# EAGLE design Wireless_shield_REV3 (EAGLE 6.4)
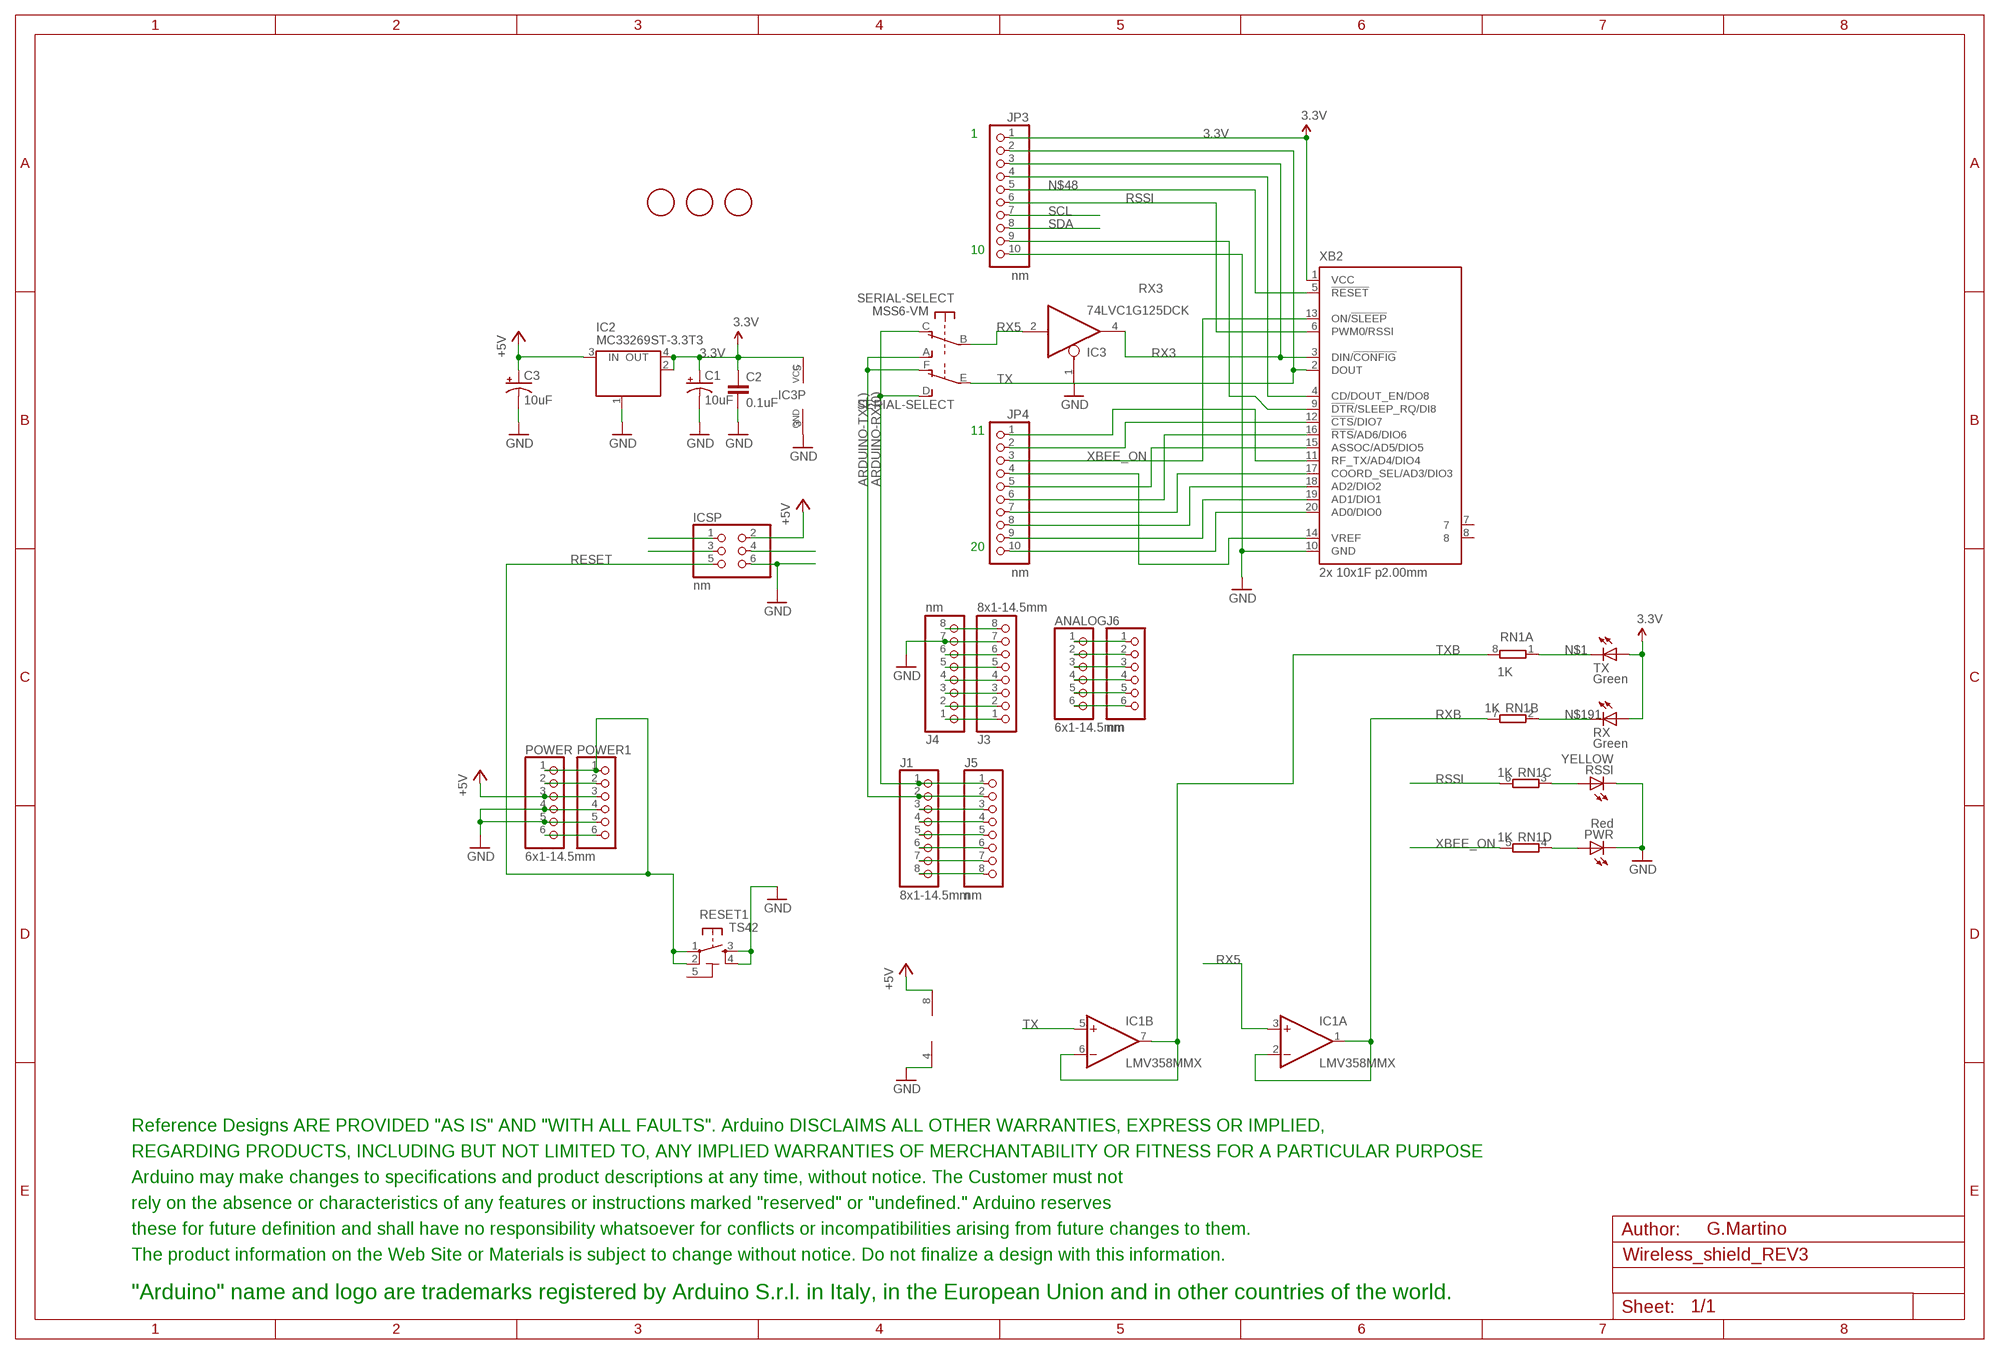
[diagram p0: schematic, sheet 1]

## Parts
A1  FIDUCIALMOUNT  [FIDUCIA-MOUNT]
A2  FIDUCIALMOUNT  [FIDUCIA-MOUNT]
A3  FIDUCIALMOUNT  [FIDUCIA-MOUNT]
ANALOG  6x1-14.5mm  PINHD-1X6  [1X06]
C1  10uF  CAP_POL1206  [EIA3216]
C2  0.1uF  CAP0603-CAP  [0603-CAP]
C3  10uF  CAP_POL1206  [EIA3216]
IC1  LMV358MMX  [MSOP08]
IC2  MC33269ST-3.3T3  [SOT223]
IC3  74LVC1G125DCK  [SC70-5]
ICSP  nm  PINHD-2X3  [2X03]
J1  8x1-14.5mm  PINHD-1X8  [1X08]
J3  8x1-14.5mm  PINHD-1X8  [1X08]
J4  nm  PINHD-1X8  [1X08]
J5  nm  PINHD-1X8  [1X08]
J6  nm  PINHD-1X6  [1X06]
JP3  nm  PINHD-1X10  [1X10]
JP4  nm  PINHD-1X10  [1X10]
POWER  6x1-14.5mm  PINHD-1X6  [1X06]
POWER1  PINHD-1X6  [1X06]
PWR  Red  LEDCHIP-LED0805  [CHIP-LED0805]
RESET1  TS42  [TS42]
RN1  1K  4R-NCAY16  [CAY16]
RSSI  YELLOW  LEDCHIP-LED0805  [CHIP-LED0805]
RX  Green  LEDCHIP-LED0805  [CHIP-LED0805]
SERIAL-SELECT  MSS6-VM  [MSS6-V]
TX  Green  LEDCHIP-LED0805  [CHIP-LED0805]
U$2  DISCLAIMER-SMALL  [DISCLAIMER]
XB2  2x 10x1F p2.00mm  XBEE-PRO  [XBEE-PRO]

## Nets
3.3V: C1.A(+) C2.1 IC2.2(OUT) IC2.4(OUT) IC3.5(VCC) JP3.1 RX.A TX.A XB2.1(VCC)
+5V: C3.A(+) IC1.8(P:V+) IC2.3(IN) ICSP.2 POWER1.3 POWER.3
ARDUINO-RX(0): J1.1 J5.1 SERIAL-SELECT.C(O) SERIAL-SELECT.D(S)
ARDUINO-TX(1): J1.2 J5.2 SERIAL-SELECT.A(S) SERIAL-SELECT.F(O)
GND: C1.C(-) C2.2 C3.C(-) IC1.4(P:V-) IC2.1(GND/ADJ) IC3.1(OE) IC3.3(GND) ICSP.6 J3.7 J4.7 JP3.10 POWER1.4 POWER1.5 POWER.4 POWER.5 PWR.C RESET1.3 RESET1.4 RSSI.C XB2.10(GND)
N$1: RN1.1 TX.C
N$2: J3.1 J4.1
N$3: ICSP.3
N$4: ICSP.1
N$5: ICSP.4
N$6: J3.2 J4.2
N$7: J3.3 J4.3
N$9: J3.6 J4.6
N$10: J1.3 J5.3
N$11: J1.4 J5.4
N$12: J1.5 J5.5
N$13: J1.6 J5.6
N$14: J1.7 J5.7
N$15: J1.8 J5.8
N$16: RN1.3 RSSI.A
N$18: ANALOG.1 J6.1
N$19: ANALOG.2 J6.2
N$20: ANALOG.3 J6.3
N$21: ANALOG.4 J6.4
N$22: ANALOG.5 J6.5
N$23: ANALOG.6 J6.6
N$24: JP4.10 XB2.20(AD0/DIO0)
N$25: JP4.9 XB2.19(AD1/DIO1)
N$27: J3.5 J4.5
N$28: JP4.8 XB2.18(AD2/DIO2)
N$29: PWR.A RN1.4
N$30: POWER1.6 POWER.6
N$33: JP4.7 XB2.17(COORD_SEL/AD3/DIO3)
N$34: JP4.6 XB2.16(!RTS!/AD6/DIO6)
N$36: JP4.5 XB2.15(ASSOC/AD5/DIO5)
N$37: JP4.4 XB2.14(VREF)
N$39: JP4.2 XB2.12(!CTS!/DIO7)
N$41: JP4.1 XB2.11(RF_TX/AD4/DIO4)
N$43: JP3.4 XB2.4(CD/DOUT_EN/DO8)
N$48: JP3.5 XB2.5(!RESET)
N$50: JP3.9 XB2.9(!DTR!/SLEEP_RQ/DI8)
N$61: J3.4 J4.4
N$191: RN1.2 RX.C
N$222: J3.8 J4.8
N$223: POWER1.2 POWER.2
RESET: ICSP.5 POWER1.1 POWER.1 RESET1.1 RESET1.2
RSSI: JP3.6 RN1.6 XB2.6(PWM0/RSSI)
RX3: IC3.4(O) JP3.3 XB2.3(DIN/!CONFIG)
RX5: IC1.3(A:+IN) IC3.2(I) SERIAL-SELECT.B(P)
RXB: IC1.1(A:OUT) IC1.2(A:-IN) RN1.7
SCL: JP3.7
SDA: JP3.8
TX: IC1.5(B:+IN) JP3.2 SERIAL-SELECT.E(P) XB2.2(DOUT)
TXB: IC1.6(B:-IN) IC1.7(B:OUT) RN1.8
XBEE_ON: JP4.3 RN1.5 XB2.13(ON/!SLEEP)
Unconnected: XB2.7 XB2.8

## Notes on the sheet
- 1
- 10
- 11
- 20
- G.Martino

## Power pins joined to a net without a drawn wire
5-GND: RESET1.5(5-GND)

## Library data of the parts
A1-A3 = Smartprj:FIDUCIALMOUNT
ANALOG J6 POWER POWER1 = pinhead:PINHD-1X6: PIN HEADER
C1 C3 = SparkFun:CAP_POL: Capacitor Polarized
C2 = SparkFun:CAP: Capacitor
IC1 = linear:LMV358?*: Dual General Purpose, Low Voltage, Rail-to-Rail Output Operational Amplifiers Source: http://www.national.com/mpf/LM/LMV321.html http://www.national.com/dt/lmv_qual.pdf
IC2 = linear:MC33269ST*: Adjustable Output Low Dropout Voltage Regulator 800 mA Source: http://www.onsemi.com/pub/Collateral/MC33269-D.PDF
IC3 = 74xx-little-us:74*1G125: Single Bus Buffer Gate with 3-State Output
ICSP = pinhead:PINHD-2X3: PIN HEADER
J1 J3-J5 = pinhead:PINHD-1X8: PIN HEADER
JP3 JP4 = pinhead:PINHD-1X10: PIN HEADER
PWR RSSI RX TX = led:LED: LED
RESET1 = st-mod v1.4:TS42: TS42 Dongnan Electronics Tact switch VDC 12V - 50mA
RN1 = resistor-dil:4R-N: Array Chip Resistor Source: RS Component / Phycomp
SERIAL-SELECT = Smartprj:MSS6-V
U$2 = Misc:DISCLAIMER-SMALL: DISCLAIMER
XB2 = maxstream:XBEE: XBee (TM) /XBee-PRO(TM) OEM RF Modules Source: MaxStream, Inc. xbee_productmanual.pdf

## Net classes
0 default: width 0.203 mm, drill 0.559 mm, clearance 0.203 mm
2 gnd: width 0.203 mm, drill 0.559 mm, clearance 0.203 mm

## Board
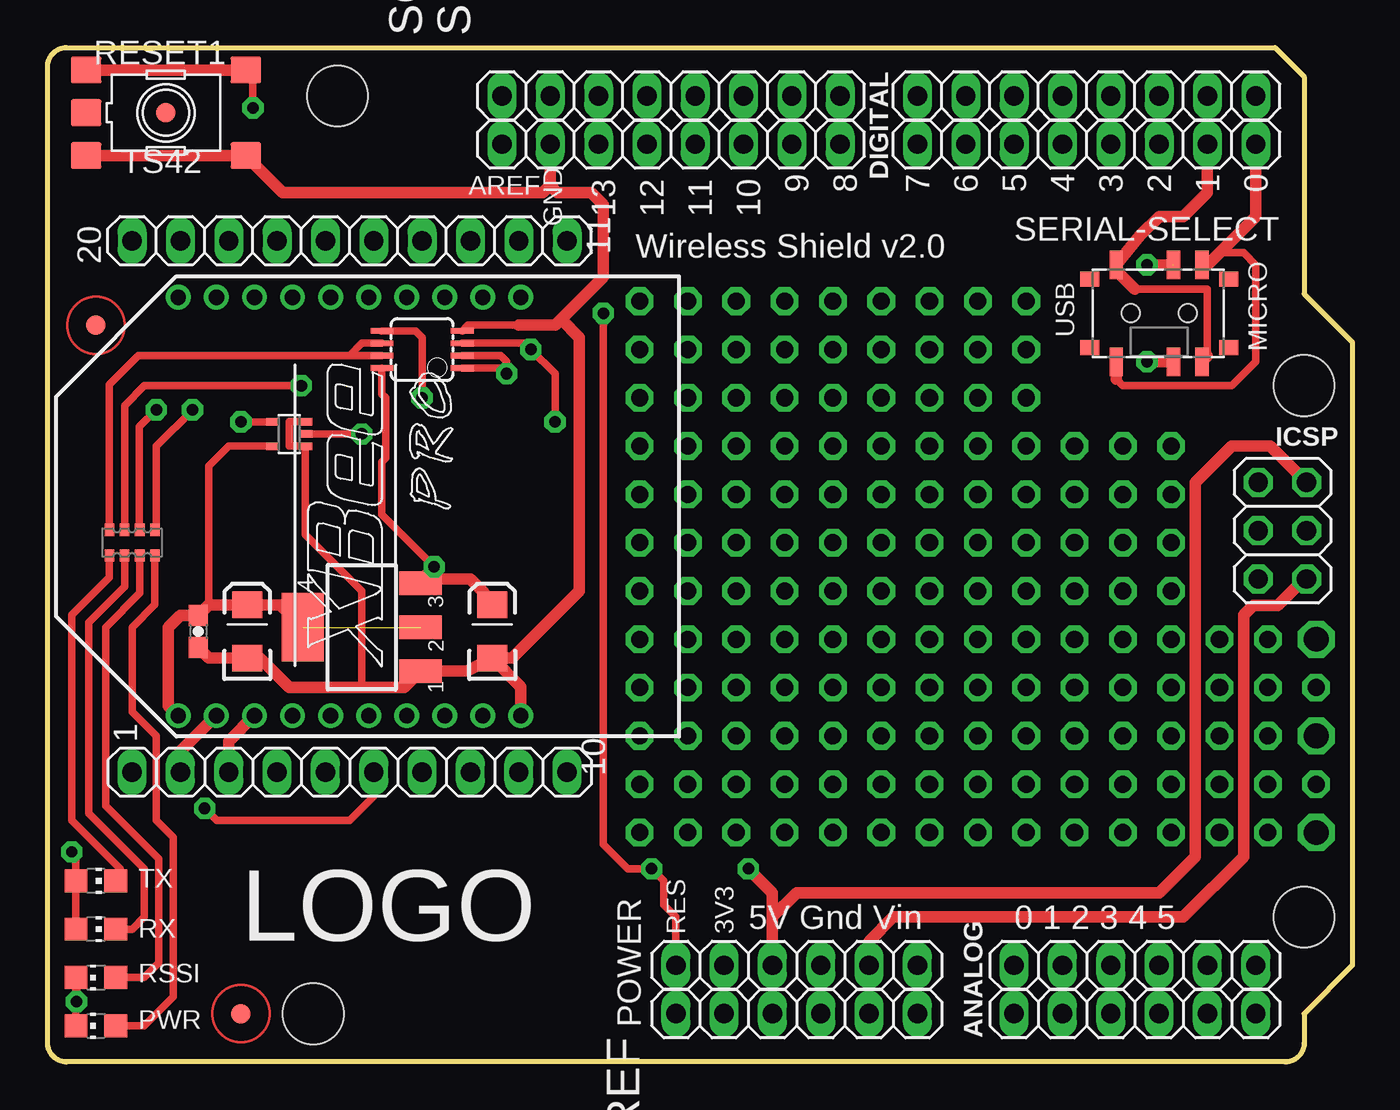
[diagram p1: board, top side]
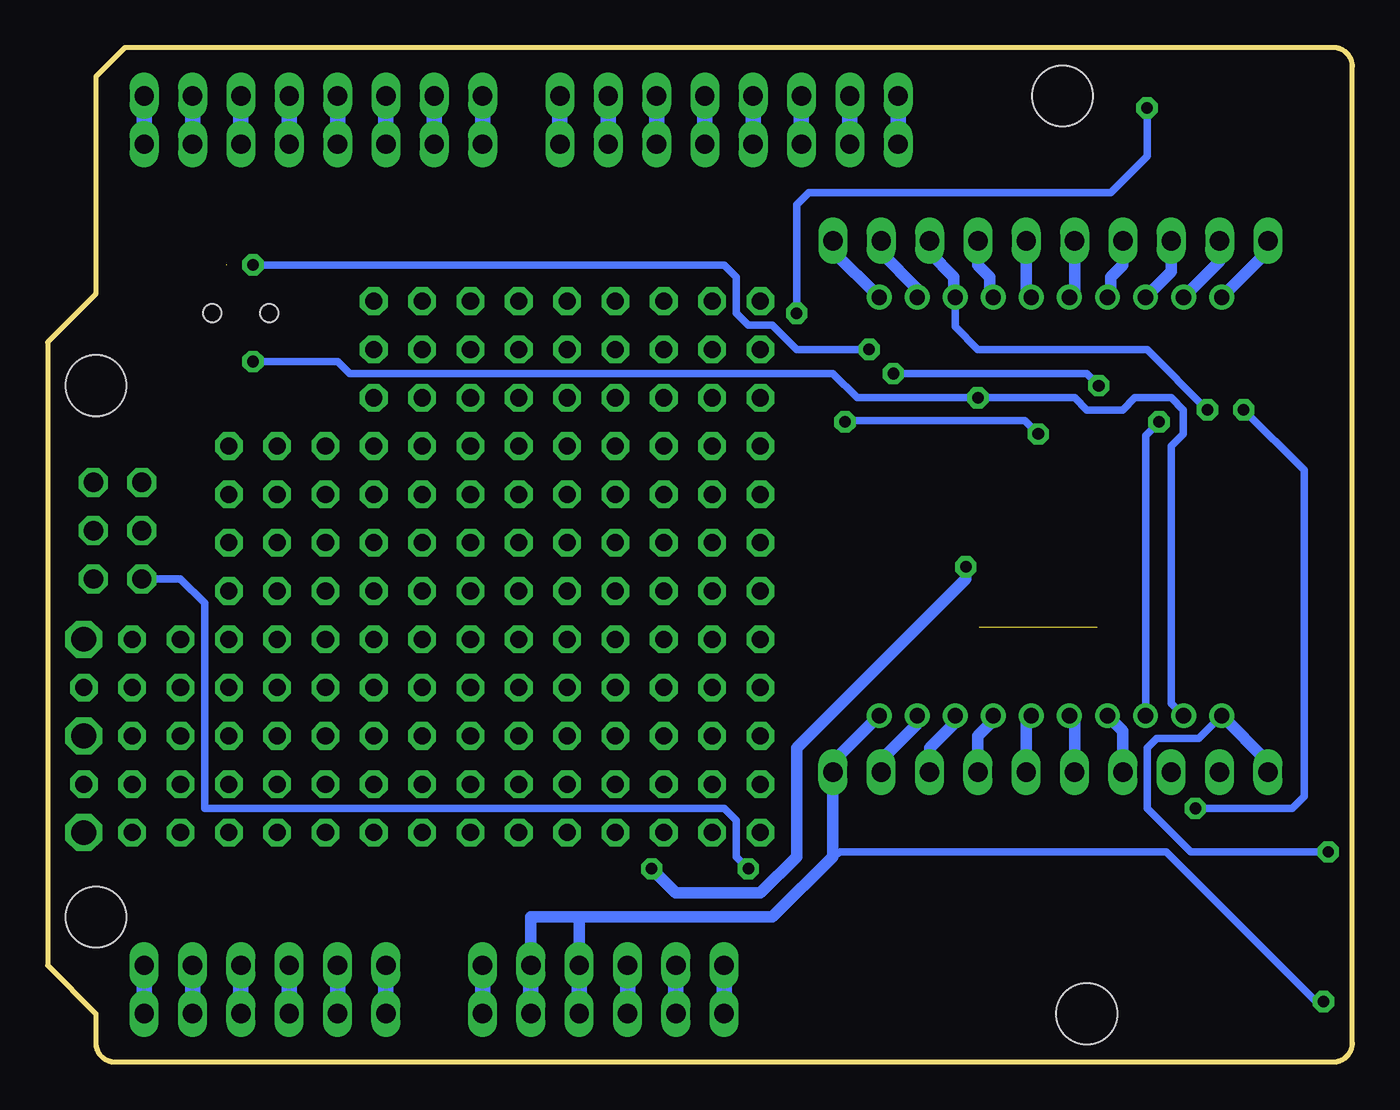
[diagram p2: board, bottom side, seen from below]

Size 68.58 x 53.34 mm. Coordinates in mm from the lower left corner, seen from the top.
Outline: 64.52,53.34 66.04,51.82 66.04,40.39 68.58,37.85 68.58,5.08 66.04,2.54 66.04,1 arc-90 65.04,0 1,0 arc-90 0,1 0,52.34 arc-90 1,53.34 64.52,53.34
Copper layers (1*16): Top 0.035mm / dielectric 1.5mm / Bottom 0.035mm
Design rules "ArduinoUno *": minimum track width 12mil, minimum drill 32mil, track to track 12mil, track to pad 12mil, pad to pad 12mil, via to via 12mil, smd to smd 12mil, copper to edge 32mil, drill to drill 16mil, minimum pad ring 10mil, minimum via ring 10mil, stop-mask expansion 2mil, vias tented up to drill 30mil, thermal gap 10mil
Holes 3.2 mm at 15.24,50.8 66.04,7.62 66.04,35.56 13.97,2.54

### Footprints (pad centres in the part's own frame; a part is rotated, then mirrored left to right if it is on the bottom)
FIDUCIA-MOUNT = smd 1.016 x 1.016: P$1 0,0
1X06 = drill 1.016 long: 1 -6.35,0; 2 -3.81,0; 3 -1.27,0; 4 1.27,0; 5 3.81,0; 6 6.35,0
EIA3216 = smd 1.4 x 1.6: A 1.4,0; C -1.4,0
0603-CAP = smd 1.1 x 1: 1 -0.85,0; 2 0.85,0
MSOP08 = smd 0.3 x 1.2: 1 -0.976,-2.113; 2 -0.326,-2.113; 3 0.324,-2.113; 4 0.974,-2.113; 5 0.974,2.112; 6 0.324,2.112; 7 -0.326,2.112; 8 -0.976,2.112
SOT223 = smd 1.219 x 2.235: 1 -2.311,-3.099; 2 0,-3.099; 3 2.311,-3.099 | smd 3.6 x 2.2: 4 0,3.099
SC70-5 = smd 0.4 x 0.7: 1 -0.65,-0.85; 2 0,-0.85; 3 0.65,-0.85; 4 0.65,0.85; 5 -0.65,0.85
2X03 = drill 1.016 octagon: 1 -2.54,-1.27; 2 -2.54,1.27; 3 0,-1.27; 4 0,1.27; 5 2.54,-1.27; 6 2.54,1.27
1X08 = drill 1.016 long: 1 -8.89,0; 2 -6.35,0; 3 -3.81,0; 4 -1.27,0; 5 1.27,0; 6 3.81,0; 7 6.35,0; 8 8.89,0
1X10 = drill 1.016 long: 1 -11.43,0; 2 -8.89,0; 3 -6.35,0; 4 -3.81,0; 5 -1.27,0; 6 1.27,0; 7 3.81,0; 8 6.35,0; 9 8.89,0; 10 11.43,0
CHIP-LED0805 = smd 1.2 x 1.2: A 0,-1.05; C 0,1.05
TS42 = smd 1.6 x 1.4: 1 -4.2,2.25; 2 4.2,2.25; 3 -4.2,-2.25; 4 4.2,-2.25; 5 -4.2,0
CAY16 = smd 0.5 x 0.65: 1 -1.2,-0.675; 2 -0.4,-0.675; 3 0.4,-0.675; 4 1.2,-0.675; 5 1.2,0.675; 6 0.4,0.675; 7 -0.4,0.675; 8 -1.2,0.675
MSS6-V = smd 1 x 0.8: 7 -3.65,1.8; 8 -3.65,-1.8; 9 3.65,1.8; 10 3.65,-1.8 | smd 0.7 x 1.5: A -2.25,2.55; B 0.75,2.55; C 2.25,2.55; D -2.25,-2.55; E 0.75,-2.55; F 2.25,-2.55 | hole 0.95: -1.5,0; 1.5,0
XBEE-PRO = drill 0.8 pad 1.27: 1 -11,9; 2 -11,7; 3 -11,5; 4 -11,3; 5 -11,1; 6 -11,-1; 7 -11,-3; 8 -11,-5; 9 -11,-7; 10 -11,-9; 11 11,-9; 12 11,-7; 13 11,-5; 14 11,-3; 15 11,-1; 16 11,1; 17 11,3; 18 11,5; 19 11,7; 20 11,9

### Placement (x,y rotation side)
A1  6.22,49.91 0 top
A2  10.16,2.54 0 top
A3  2.54,38.73 0 top
ANALOG  57.15,2.54 0 top
C1  10.49,22.64 90 top
C2  7.92,22.64 270 top
C3  23.37,22.64 90 top
IC1  19.68,37.47 90 top
IC2  16.51,22.86 90 top
IC3  12.7,33.02 90 top
ICSP  64.9,27.94 270 top
J1  54.61,50.8 180 top
J3  32.77,50.8 180 top
J4  32.77,48.26 180 top
J5  54.61,48.26 180 top
J6  57.15,5.08 0 top
JP3  15.88,15.24 0 top
JP4  15.88,43.18 180 top
POWER  39.37,2.54 0 top
POWER1  39.37,5.08 0 top
PWR  2.54,1.91 90 top
RESET1  6.22,49.91 0 top
RN1  4.45,27.3 0 top
RSSI  2.54,4.45 90 top
RX  2.54,6.99 270 top
SERIAL-SELECT  58.42,39.37 0 top
TX  2.54,9.53 270 top
U$2  not placed on the board
XB2  15.88,29.21 90 top

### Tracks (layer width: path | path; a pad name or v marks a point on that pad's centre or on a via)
3.3V  (via drill 0.6)  (1 unrouted)
  Top 0.406: RX.A TX.A 1.49,10.57 v1.27,11.05 | 8.46,24.04 8.46,31.32 9.53,32.38 11.84,32.38 IC3.5
  Top 0.61: XB2.1 6.35,18.72 6.35,22.86 6.97,23.48 C2.1 8.46,24.04 C1.A 12.24,24.04 IC2.4
  Bottom 0.406: v1.27,11.05 8.51,11.05 10.79,13.34 10.79,16.51 10.29,17.02 8.07,17.02 XB2.1
  Bottom 0.61: JP3.1 4.45,15.78 XB2.1
+5V  (via drill 0.61)
  Top 0.406: IC1.8 17.57,35.13 17.78,34.92 17.78,31.75 17.57,31.54 17.57,28.78 v20.32,26.04
  Top 0.61: 38.1,7.62 POWER1.3 | 38.1,7.62 39.37,8.89 58.42,8.89 60.33,10.79 60.33,30.48 62.23,32.38 64.26,32.38 ICSP.2 | 38.1,7.62 38.1,8.89 v36.83,10.16 | C3.A 22.95,24.67 22.23,25.4 19.84,25.4 | 19.84,25.4 IC2.3 | 19.84,25.4 19.84,25.55 v20.32,26.04
  Bottom 0.61: v36.83,10.16 35.56,8.89 31.11,8.89 29.21,10.79 29.21,16.51 20.32,25.4 v20.32,26.04
  Bottom 0.813: POWER1.3 POWER.3
ARDUINO-RX(0)
  Top 0.406: 56.17,35.91 56.52,35.56 62.23,35.56 63.5,36.83 63.5,41.91 62.87,42.55 61.59,42.55 61.28,42.23
  Top 0.61: J5.1 63.5,44.45 61.28,42.23 60.97,41.92 SERIAL-SELECT.C | SERIAL-SELECT.D 56.17,35.91
  Bottom 0.813: J5.1 J1.1
ARDUINO-TX(1)
  Top 0.406: 56.17,41.62 SERIAL-SELECT.A | 57.15,40.64 60.96,40.64 60.96,37.11
  Top 0.61: SERIAL-SELECT.A 57.44,43.47 58.42,44.45 59.69,44.45 60.96,45.72 J5.2 | 57.15,40.64 56.17,41.62 | SERIAL-SELECT.F 60.96,37.11
  Bottom 0.813: J5.2 J1.2
GND  (via drill 0.61)
  Top 0.406: PWR.C RSSI.C 1.52,4.41 v1.52,3.17 | 24.77,38.73 22.09,38.73 IC1.4 | IC3.3 12.71,33.67 12.7,33.66 12.7,32.38 13.54,32.38 IC3.1 13.55,27.73 16.51,24.77 16.51,19.68
  Top 0.61: RESET1.3 RESET1.4 12.36,45.72 26.04,45.72 26.42,46.1 | C2.2 8.46,21.23 C1.C 11.15,21.23 12.7,19.68 16.51,19.68 18.75,19.68 IC2.1 22.05,20.55 C3.C | 26.42,46.1 J4.7 | 24.77,38.73 26.67,38.73 26.99,39.05 | 26.99,39.05 29.21,41.27 29.21,45.09 28.57,45.72 26.8,45.72 26.42,46.1 | 26.99,39.05 27.94,38.1 27.94,24.77 24.41,21.23 C3.C | ICSP.6 66.04,25.4 64.64,24 63.37,24 62.87,23.5 62.87,10.79 59.69,7.62 44.45,7.62 43.18,6.35 POWER1.5 | XB2.10 24.88,19.73 C3.C
  Bottom 0.406: v1.52,3.17 1.91,3.17 9.78,11.05 26.92,11.05 27.3,10.79
  Bottom 0.61: XB2.10 27.3,15.78 JP3.10 27.3,10.79 30.48,7.62 40.64,7.62 | 40.64,7.62 POWER1.4 | POWER1.5 43.18,7.62 40.64,7.62
  Bottom 0.813: J4.7 J3.7 | POWER1.4 POWER.4 | POWER1.5 POWER.5
N$1
  Top 0.406: RN1.1 3.25,25.47 1.27,23.5 1.27,12.7 3.81,10.16 3.81,9.74 TX.C
N$2
  Bottom 0.813: J4.1 J3.1
N$6
  Bottom 0.813: J4.2 J3.2
N$7
  Bottom 0.813: J4.3 J3.3
N$8  (via drill 0.9 pad 1.45)
  other vias: 33.66,32.38
N$9
  Bottom 0.813: J4.6 J3.6
N$10
  Bottom 0.813: J1.3 J5.3 58.42,47.62
N$11
  Bottom 0.813: J5.4 J1.4
N$12
  Bottom 0.813: J5.5 J1.5
N$13
  Bottom 0.813: J5.6 J1.6
N$14
  Bottom 0.813: J5.7 J1.7
N$15
  Bottom 0.813: J5.8 J1.8
N$16
  Top 0.406: RSSI.A 5.08,4.45 5.84,5.21 5.84,10.67 3.05,13.46 3.05,22.86 4.84,24.66 RN1.3
N$17  (via drill 0.9 pad 1.45)
  other vias: 59.05,19.68
N$18
  Bottom 0.813: ANALOG.1 J6.1
N$19
  Bottom 0.813: ANALOG.2 J6.2
N$20
  Bottom 0.813: ANALOG.3 J6.3
N$21
  Bottom 0.813: ANALOG.4 J6.4
N$22
  Bottom 0.813: ANALOG.5 J6.5
N$23
  Bottom 0.813: ANALOG.6 J6.6
N$24
  Bottom 0.61: JP4.10 4.45,42.64 XB2.20
N$25
  Bottom 0.61: JP4.9 6.99,42.1 XB2.19
N$27
  Bottom 0.813: J4.5 J3.5
N$28
  Bottom 0.61: JP4.8 9.53,41.56 XB2.18
N$29
  Top 0.406: PWR.A 5.08,1.91 6.6,3.43 6.6,11.81 5.71,12.7 5.71,17.14 4.45,18.41 4.45,22.86 5.64,24.06 RN1.4
N$30
  Bottom 0.813: POWER.6 POWER1.6
N$31  (via drill 1.3 pad 1.93)
  other vias: 66.67,17.14
N$32  (via drill 0.9 pad 1.45)
  other vias: 33.66,40.01
N$33
  Bottom 0.61: JP4.7 12.06,41.91 12.7,41.27 12.7,40.38 XB2.17
N$34
  Bottom 0.61: JP4.6 14.61,40.48 XB2.16
N$35  (via drill 0.9 pad 1.45)
  other vias: 33.66,37.47
N$36
  Bottom 0.61: JP4.5 17.14,40.48 XB2.15
N$37
  Bottom 0.61: JP4.4 19.68,41.91 19.05,41.27 19.05,40.38 XB2.14
N$38  (via drill 0.9 pad 1.45)
  other vias: 33.66,34.92
N$39
  Bottom 0.61: JP4.2 24.77,42.55 22.86,40.64 22.86,40.23 XB2.12
N$40  (via drill 0.9 pad 1.45)
  other vias: 59.05,14.61
N$41
  Bottom 0.61: JP4.1 27.3,42.64 XB2.11
N$42  (via drill 0.9 pad 1.45)
  other vias: 59.05,27.3
N$43
  Bottom 0.61: JP3.4 12.06,17.4 XB2.4
N$44  (via drill 1.3 pad 1.93)
  other vias: 66.67,22.23
N$45  (via drill 0.9 pad 1.45)
  other vias: 66.67,19.68
N$46  (via drill 0.9 pad 1.45)
  other vias: 59.05,24.77
N$47  (via drill 0.9 pad 1.45)
  other vias: 59.05,22.23
N$48
  Bottom 0.61: JP3.5 14.61,17.94 XB2.5
N$49  (via drill 0.9 pad 1.45)
  other vias: 66.67,14.61
N$50
  Bottom 0.61: JP3.9 24.77,15.88 22.86,17.78 22.86,18.2 XB2.9
N$51  (via drill 0.9 pad 1.45)
  other vias: 61.59,22.23
N$52  (via drill 0.9 pad 1.45)
  other vias: 59.05,17.14
N$53  (via drill 0.9 pad 1.45)
  other vias: 61.59,17.14
N$54  (via drill 0.9 pad 1.45)
  other vias: 59.05,12.06
N$55  (via drill 0.9 pad 1.45)
  other vias: 33.66,29.84
N$56  (via drill 0.9 pad 1.45)
  other vias: 61.59,12.06
N$57  (via drill 0.9 pad 1.45)
  other vias: 33.66,27.3
N$58  (via drill 0.9 pad 1.45)
  other vias: 33.66,24.77
N$59  (via drill 1.3 pad 1.93)
  other vias: 66.67,12.06
N$60  (via drill 0.9 pad 1.45)
  other vias: 48.9,40.01
N$61
  Bottom 0.813: J4.4 J3.4
N$62  (via drill 0.9 pad 1.45)
  other vias: 43.81,40.01
N$63  (via drill 0.9 pad 1.45)
  other vias: 33.66,22.23
N$64  (via drill 0.9 pad 1.45)
  other vias: 38.73,40.01
N$65  (via drill 0.9 pad 1.45)
  other vias: 33.66,19.68
N$66  (via drill 0.9 pad 1.45)
  other vias: 33.66,17.14
N$67  (via drill 0.9 pad 1.45)
  other vias: 33.66,14.61
N$68  (via drill 0.9 pad 1.45)
  other vias: 33.66,12.06
N$69  (via drill 0.9 pad 1.45)
  other vias: 31.11,32.38
N$70  (via drill 0.9 pad 1.45)
  other vias: 31.11,29.84
N$71  (via drill 0.9 pad 1.45)
  other vias: 31.11,27.3
N$72  (via drill 0.9 pad 1.45)
  other vias: 31.11,24.77
N$73  (via drill 0.9 pad 1.45)
  other vias: 61.59,19.68
N$74  (via drill 0.9 pad 1.45)
  other vias: 51.44,40.01
N$75  (via drill 0.9 pad 1.45)
  other vias: 31.11,22.23
N$76  (via drill 0.9 pad 1.45)
  other vias: 41.27,40.01
N$77  (via drill 0.9 pad 1.45)
  other vias: 36.2,40.01
N$78  (via drill 0.9 pad 1.45)
  other vias: 61.59,14.61
N$79  (via drill 0.9 pad 1.45)
  other vias: 48.9,37.47
N$80  (via drill 0.9 pad 1.45)
  other vias: 43.81,37.47
N$81  (via drill 0.9 pad 1.45)
  other vias: 38.73,37.47
N$82  (via drill 0.9 pad 1.45)
  other vias: 31.11,19.68
N$83  (via drill 0.9 pad 1.45)
  other vias: 59.05,29.84
N$84  (via drill 0.9 pad 1.45)
  other vias: 51.44,37.47
N$85  (via drill 0.9 pad 1.45)
  other vias: 46.35,40.01
N$86  (via drill 0.9 pad 1.45)
  other vias: 41.27,37.47
N$87  (via drill 0.9 pad 1.45)
  other vias: 36.2,37.47
N$88  (via drill 0.9 pad 1.45)
  other vias: 59.05,32.38
N$89  (via drill 0.9 pad 1.45)
  other vias: 48.9,34.92
N$90  (via drill 0.9 pad 1.45)
  other vias: 43.81,34.92
N$91  (via drill 0.9 pad 1.45)
  other vias: 38.73,34.92
N$92  (via drill 0.9 pad 1.45)
  other vias: 31.11,17.14
N$93  (via drill 0.9 pad 1.45)
  other vias: 64.14,19.68
N$94  (via drill 0.9 pad 1.45)
  other vias: 51.44,34.92
N$95  (via drill 0.9 pad 1.45)
  other vias: 46.35,34.92
N$96  (via drill 0.9 pad 1.45)
  other vias: 41.27,34.92
N$97  (via drill 0.9 pad 1.45)
  other vias: 36.2,34.92
N$98  (via drill 0.9 pad 1.45)
  other vias: 53.98,32.38
N$99  (via drill 0.9 pad 1.45)
  other vias: 48.9,32.38
N$100  (via drill 0.9 pad 1.45)
  other vias: 43.81,32.38
N$101  (via drill 0.9 pad 1.45)
  other vias: 38.73,32.38
N$102  (via drill 0.9 pad 1.45)
  other vias: 31.11,14.61
N$103  (via drill 0.9 pad 1.45)
  other vias: 56.52,32.38
N$104  (via drill 0.9 pad 1.45)
  other vias: 51.44,32.38
N$105  (via drill 0.9 pad 1.45)
  other vias: 46.35,32.38
N$106  (via drill 0.9 pad 1.45)
  other vias: 41.27,32.38
N$107  (via drill 0.9 pad 1.45)
  other vias: 36.2,32.38
N$108  (via drill 0.9 pad 1.45)
  other vias: 53.98,29.84
N$109  (via drill 0.9 pad 1.45)
  other vias: 48.9,29.84
N$110  (via drill 0.9 pad 1.45)
  other vias: 43.81,29.84
N$111  (via drill 0.9 pad 1.45)
  other vias: 38.73,29.84
N$112  (via drill 0.9 pad 1.45)
  other vias: 31.11,12.06
N$113  (via drill 0.9 pad 1.45)
  other vias: 56.52,29.84
N$114  (via drill 0.9 pad 1.45)
  other vias: 51.44,29.84
N$115  (via drill 0.9 pad 1.45)
  other vias: 46.35,29.84
N$116  (via drill 0.9 pad 1.45)
  other vias: 41.27,29.84
N$117  (via drill 0.9 pad 1.45)
  other vias: 36.2,29.84
N$118  (via drill 0.9 pad 1.45)
  other vias: 53.98,27.3
N$119  (via drill 0.9 pad 1.45)
  other vias: 48.9,27.3
N$120  (via drill 0.9 pad 1.45)
  other vias: 43.81,27.3
N$121  (via drill 0.9 pad 1.45)
  other vias: 38.73,27.3
N$122  (via drill 0.9 pad 1.45)
  other vias: 31.11,40.01
N$123  (via drill 0.9 pad 1.45)
  other vias: 56.52,27.3
N$124  (via drill 0.9 pad 1.45)
  other vias: 51.44,27.3
N$125  (via drill 0.9 pad 1.45)
  other vias: 46.35,27.3
N$126  (via drill 0.9 pad 1.45)
  other vias: 41.27,27.3
N$127  (via drill 0.9 pad 1.45)
  other vias: 36.2,27.3
N$128  (via drill 0.9 pad 1.45)
  other vias: 53.98,24.77
N$129  (via drill 0.9 pad 1.45)
  other vias: 48.9,24.77
N$130  (via drill 0.9 pad 1.45)
  other vias: 43.81,24.77
N$131  (via drill 0.9 pad 1.45)
  other vias: 38.73,24.77
N$132  (via drill 0.9 pad 1.45)
  other vias: 31.11,37.47
N$133  (via drill 0.9 pad 1.45)
  other vias: 56.52,24.77
N$134  (via drill 0.9 pad 1.45)
  other vias: 51.44,24.77
N$135  (via drill 0.9 pad 1.45)
  other vias: 46.35,24.77
N$136  (via drill 0.9 pad 1.45)
  other vias: 41.27,24.77
N$137  (via drill 0.9 pad 1.45)
  other vias: 36.2,24.77
N$138  (via drill 0.9 pad 1.45)
  other vias: 53.98,22.23
N$139  (via drill 0.9 pad 1.45)
  other vias: 48.9,22.23
N$140  (via drill 0.9 pad 1.45)
  other vias: 43.81,22.23
N$141  (via drill 0.9 pad 1.45)
  other vias: 38.73,22.23
N$142  (via drill 0.9 pad 1.45)
  other vias: 31.11,34.92
N$143  (via drill 0.9 pad 1.45)
  other vias: 56.52,22.23
N$144  (via drill 0.9 pad 1.45)
  other vias: 51.44,22.23
N$145  (via drill 0.9 pad 1.45)
  other vias: 46.35,22.23
N$146  (via drill 0.9 pad 1.45)
  other vias: 41.27,22.23
N$147  (via drill 0.9 pad 1.45)
  other vias: 36.2,22.23
N$148  (via drill 0.9 pad 1.45)
  other vias: 53.98,19.68
N$149  (via drill 0.9 pad 1.45)
  other vias: 48.9,19.68
N$150  (via drill 0.9 pad 1.45)
  other vias: 43.81,19.68
N$151  (via drill 0.9 pad 1.45)
  other vias: 38.73,19.68
N$152  (via drill 0.9 pad 1.45)
  other vias: 46.35,37.47
N$153  (via drill 0.9 pad 1.45)
  other vias: 56.52,19.68
N$154  (via drill 0.9 pad 1.45)
  other vias: 51.44,19.68
N$155  (via drill 0.9 pad 1.45)
  other vias: 46.35,19.68
N$156  (via drill 0.9 pad 1.45)
  other vias: 41.27,19.68
N$157  (via drill 0.9 pad 1.45)
  other vias: 36.2,19.68
N$158  (via drill 0.9 pad 1.45)
  other vias: 53.98,17.14
N$159  (via drill 0.9 pad 1.45)
  other vias: 48.9,17.14
N$160  (via drill 0.9 pad 1.45)
  other vias: 43.81,17.14
N$161  (via drill 0.9 pad 1.45)
  other vias: 38.73,17.14
N$162  (via drill 0.9 pad 1.45)
  other vias: 64.14,22.23
N$163  (via drill 0.9 pad 1.45)
  other vias: 56.52,17.14
N$164  (via drill 0.9 pad 1.45)
  other vias: 51.44,17.14
N$165  (via drill 0.9 pad 1.45)
  other vias: 46.35,17.14
N$166  (via drill 0.9 pad 1.45)
  other vias: 41.27,17.14
N$167  (via drill 0.9 pad 1.45)
  other vias: 36.2,17.14
N$168  (via drill 0.9 pad 1.45)
  other vias: 53.98,14.61
N$169  (via drill 0.9 pad 1.45)
  other vias: 48.9,14.61
N$170  (via drill 0.9 pad 1.45)
  other vias: 43.81,14.61
N$171  (via drill 0.9 pad 1.45)
  other vias: 38.73,14.61
N$172  (via drill 0.9 pad 1.45)
  other vias: 64.14,14.61
N$173  (via drill 0.9 pad 1.45)
  other vias: 56.52,14.61
N$174  (via drill 0.9 pad 1.45)
  other vias: 51.44,14.61
N$175  (via drill 0.9 pad 1.45)
  other vias: 46.35,14.61
N$176  (via drill 0.9 pad 1.45)
  other vias: 41.27,14.61
N$177  (via drill 0.9 pad 1.45)
  other vias: 36.2,14.61
N$178  (via drill 0.9 pad 1.45)
  other vias: 53.98,12.06
N$179  (via drill 0.9 pad 1.45)
  other vias: 48.9,12.06
N$180  (via drill 0.9 pad 1.45)
  other vias: 43.81,12.06
N$181  (via drill 0.9 pad 1.45)
  other vias: 38.73,12.06
N$182  (via drill 0.9 pad 1.45)
  other vias: 64.14,17.14
N$183  (via drill 0.9 pad 1.45)
  other vias: 56.52,12.06
N$184  (via drill 0.9 pad 1.45)
  other vias: 51.44,12.06
N$185  (via drill 0.9 pad 1.45)
  other vias: 46.35,12.06
N$186  (via drill 0.9 pad 1.45)
  other vias: 41.27,12.06
N$187  (via drill 0.9 pad 1.45)
  other vias: 36.2,12.06
N$188
  Bottom 0.61: 18.92,18.16 18.92,17.91 19.68,17.14 19.68,15.88
N$189  (via drill 0.9 pad 1.45)
  other vias: 64.14,12.06
N$190
  Bottom 0.61: 20.83,18.16 20.83,17.91 22.23,16.51 22.23,15.88
N$191
  Top 0.406: RX.C 4.45,6.99 5.08,7.62 5.08,10.16 2.16,13.08 2.16,23.11 4.04,25 RN1.2
N$222
  Bottom 0.813: J4.8 J3.8
N$223
  Bottom 0.813: POWER.2 POWER1.2
RESET  (via drill 0.61)
  Top 0.406: POWER1.1 33.02,7.62 32.38,8.26 32.38,9.53 v31.75,10.16 30.48,10.16 29.21,11.43 v29.21,39.37 | RESET1.2 10.79,51.79 v10.79,50.16
  Top 0.61: RESET1.2 RESET1.1
  Bottom 0.406: ICSP.5 61.59,25.4 60.33,24.13 60.33,13.34 33.02,13.34 32.38,12.7 32.38,10.79 v31.75,10.16 | v10.79,50.16 10.79,47.62 12.7,45.72 28.57,45.72 29.21,45.09 v29.21,39.37
  Bottom 0.813: POWER.1 POWER1.1
RSSI  (via drill 0.61)
  Top 0.406: RN1.6 4.83,27.96 4.83,33.4 v5.71,34.29 | JP3.6 17.14,13.97 15.88,12.7 8.89,12.7 v8.26,13.34
  Bottom 0.406: v8.26,13.34 3.17,13.34 2.54,13.97 2.54,31.11 v5.71,34.29
  Bottom 0.61: JP3.6 17.14,17.94 XB2.6
RX3  (via drill 0.61)
  Top 0.406: v10.16,33.66 11.84,33.66 IC3.4
  Top 0.61: JP3.3 9.53,16.86 XB2.3
  Bottom 0.406: XB2.3 10.88,32.94 v10.16,33.66
RX5  (via drill 0.61)  (1 unrouted)
  Top 0.406: v26.67,33.66 26.67,36.2 v25.4,37.47 25.08,37.79 IC1.3 | IC3.2 v16.51,33.02
  Top 0.61: v57.78,41.91 SERIAL-SELECT.B
  Bottom 0.406: v57.78,41.91 33.02,41.91 32.38,41.27 32.38,39.37 31.75,38.73 30.48,38.73 29.21,37.47 v25.4,37.47 | v26.67,33.66 26.11,33.73 17.23,33.73 v16.51,33.02
RXB  (via drill 0.61)
  Top 0.406: RN1.7 4.04,34.52 5.08,35.56 v13.34,35.56 | IC1.2 23.82,37.14 24.13,36.83 v24.13,36.2 23.84,36.49 IC1.1
  Bottom 0.406: v24.13,36.2 13.97,36.2 v13.34,35.56
TX  (via drill 0.61)
  Top 0.406: IC1.5 19.35,38.44 19.68,38.1 v19.68,34.92
  Top 0.61: JP3.2 6.99,16.32 XB2.2 | SERIAL-SELECT.E 57.8,36.82 v57.78,36.83
  Bottom 0.406: XB2.2 9.53,18.86 9.53,32.38 8.89,33.02 8.89,34.29 9.53,34.92 11.43,34.92 12.06,34.29 13.97,34.29 14.61,34.92 v19.68,34.92 26.04,34.92 27.3,36.2 52.7,36.2 53.34,36.83 v57.78,36.83
TXB
  Top 0.406: RN1.8 3.25,35.63 4.75,37.14 15.88,37.14 | 15.88,37.14 IC1.7 | IC1.6 16.52,37.79 15.88,37.14
XBEE_ON  (via drill 0.61)
  Top 0.406: RN1.5 5.71,28.05 5.71,32.38 v7.62,34.29
  Bottom 0.406: v7.62,34.29 10.79,37.47 19.68,37.47 20.88,38.66 XB2.13
  Bottom 0.61: JP4.3 22.23,42.55 20.95,41.27 20.95,40.29 XB2.13

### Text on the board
tPlace: SCL | SDA | 9 | 8 | 7 | 6 | 5 | 4 | 3 | 2 | 1 | 0 | 13 | 12 | 11 | 10 | Wireless Shield v2.0 | LOGO | IOREF
tNames: DIGITAL | AREF | GND | 20 | 11 | USB | MICRO | 1 | 10 | RES | 3V3 | 5V Gnd Vin | 0 1 2 3 4 5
